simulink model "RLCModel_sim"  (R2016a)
settings: Solver=FixedStepAuto  StartTime=0.0  StopTime=Endtime  FixedStep=1e-3  RelTol=1e-3
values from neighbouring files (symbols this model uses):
  C = 100e-6    (= 0.0001)    [RLCModel.m]    (also in TankModel.m = 0.196349540849; TempModel.m = 4187; NonlinearTankModel.m = 0.196349540849; TankModel_with_Sensor.m = 0.196349540849)
  L = 100e-3    (= 0.1)    [RLCModel.m]    (also in DCMotorDisk.m = 0.2)
  R = 100    [RLCModel.m]    (also in DCMotorDisk.m = 5.7; TankModel.m = 500; TempModel.m = 0.1; TankModel_with_Sensor.m = 500)
  v = 5    [RLCModel.m]

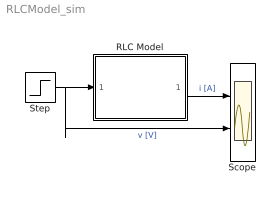
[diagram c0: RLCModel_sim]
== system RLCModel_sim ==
  RLC Model : Subsystem
  Scope : Scope  NumInputPorts=2
  Step : Step  Time=0.1  After=v  SampleTime=0
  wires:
  Step/1 -> RLC Model/1(v [V]), Scope/2  "v [V]"
  RLC Model/1(i [A]) -> Scope/1  "i [A]"

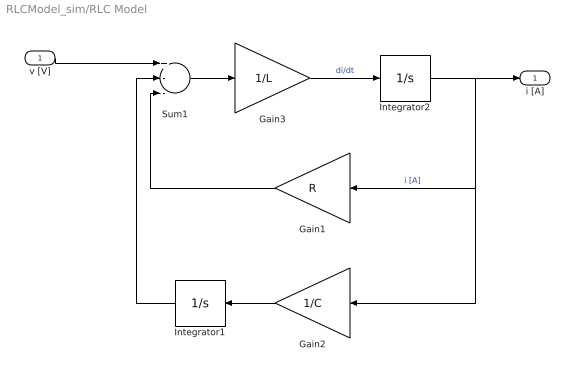
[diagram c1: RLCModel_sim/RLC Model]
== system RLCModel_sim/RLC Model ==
  v [V] : Inport
  Gain1 : Gain  Gain=R
  Gain2 : Gain  Gain=1/C
  Gain3 : Gain  Gain=1/L
  Integrator1 : Integrator
  Integrator2 : Integrator
  Sum1 : Sum  Inputs=+--
  i [A] : Outport
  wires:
  v [V]/1 -> Sum1/1
  Sum1/1 -> Gain3/1
  Gain3/1 -> Integrator2/1  "di/dt"
  Gain1/1 -> Sum1/3
  Integrator2/1 -> Gain1/1, Gain2/1, i [A]/1  "i [A]"
  Gain2/1 -> Integrator1/1
  Integrator1/1 -> Sum1/2
